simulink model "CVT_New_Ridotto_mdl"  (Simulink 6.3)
settings: Solver=ode45  StartTime=0.0  StopTime=10.0  RelTol=1e-3
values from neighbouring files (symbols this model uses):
  bt_th = -double(SysN.A)    [CVT_New.m]    (also in CVT_New_th.m = strrep(char(bt_th),'^','.^'))
  Jt_th = double(SysN.L)    [CVT_New.m]    (also in CVT_New_th.m = strrep(char(Jt_th),'^','.^'))
  Tc = 0.05*ms    (= 5e-05)    [architetture_epicicloidale_statico.m]    (also in architetture_HEV_startstop_1.m; architetture_HEV_startstop_2.m; CVT_New.m; CVT_New_th.m)
  Tt = double(SysN.Ci)    [CVT_New.m]    (also in CVT_New_th.m = Tt_t(1,:)')
  Wm_0 = 1*rpm    (= 0.10471975512)    [CVT_New.m]    (also in CVT_New_th.m)

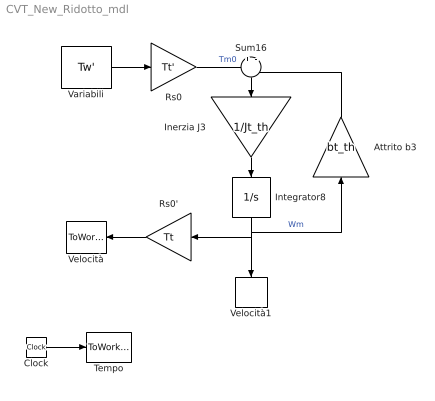
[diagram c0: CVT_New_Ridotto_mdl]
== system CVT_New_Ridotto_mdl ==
  Attrito b3 : Gain  Orientation=up  Gain=bt_th
  Clock : Clock
  Inerzia J3 : Gain  Orientation=down  Gain=1/Jt_th
  Integrator8 : Integrator  Orientation=down  InitialCondition=Wm_0  LowerSaturationLimit=0
  Rs0 : Gain  Gain=Tt'  Multiplication=Matrix(K*u)
  Rs0' : Gain  Orientation=left  Gain=Tt  Multiplication=Matrix(K*u)
  Sum16 : Sum  Orientation=down  Inputs=+|-
  Tempo : ToWorkspace  VariableName=t  SampleTime=Tc  SaveFormat=Array
  Variabili : Constant  Value=Tw'
  Velocità : ToWorkspace  VariableName=Xt  SampleTime=Tc  SaveFormat=Array
  Velocità1 : ToWorkspace  VariableName=Wm  SampleTime=Tc  SaveFormat=Array
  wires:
  Clock/1 -> Tempo/1
  Rs0/1 -> Sum16/1  "Tm0"
  Sum16/1 -> Inerzia J3/1
  Inerzia J3/1 -> Integrator8/1
  Integrator8/1 -> Rs0'/1, Attrito b3/1, Velocità1/1  "Wm"
  Attrito b3/1 -> Sum16/2
  Variabili/1 -> Rs0/1
  Rs0'/1 -> Velocità/1
